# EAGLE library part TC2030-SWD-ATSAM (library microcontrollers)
TAG-CONNECT ICSP Connector Manufacturer: Tag-Connect Cable for easy In-Circuit Serial Programming. Designed for Microchip ICD2, suitable for many others. Two variants - one "with legs" (for hands-free fit on PCB) and another "without legs" for quick programming. PADDescription 1MCLR/Vpp 2Vdd 3GND 4PGD (ISPDAT) 5PGC (ISPCLK) 6nc (used for LVP) ©2009 ROFA.cz - modified and updated by Robert Darlington &#8249;rdarlington@gmail.com&#8250;
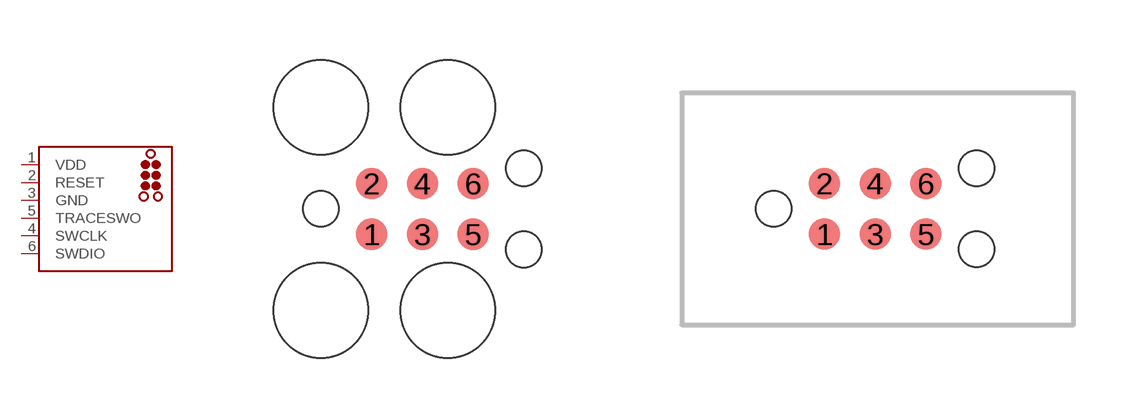
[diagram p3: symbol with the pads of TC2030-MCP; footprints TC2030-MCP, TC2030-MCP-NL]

Designator prefix J

## TC2030-SWD-ATSAM-MCP  [TC2030-MCP]
1  VDD  pwr
2  RESET  pwr
3  GND  pwr
4  SWCLK  in
5  TRACESWO  pwr
6  SWDIO

## TC2030-SWD-ATSAM-MCP-NL  [TC2030-MCP-NL]
Pads as for TC2030-MCP

## TC2030-SWD-ATSAM  [TC2030-MCP-NL-CP]
Pads as for TC2030-MCP

## Footprint TC2030-MCP (pad centres in mm)
TAG-CONNECT ICSP Connector - Legged version Manufacturer: Tag-Connect Cable for easy In-Circuit Serial Programming. Designed for Microchip ICD2, suitable for many others. NOTE: Eagle's default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
smd 0.787 x 0.787: 1 1.27,-0.635; 2 1.27,0.635; 3 2.54,-0.635; 4 2.54,0.635; 5 3.81,-0.635; 6 3.81,0.635
hole 0.889 at 0,0
hole 0.889 at 5.08,-1.016
hole 0.889 at 5.08,1.016
hole 2.375 at 0,2.54
hole 2.375 at 0,-2.54
hole 2.375 at 3.175,-2.54
hole 2.375 at 3.175,2.54

## Footprint TC2030-MCP-NL (pad centres in mm)
TAG-CONNECT ICSP Connector Manufacturer: Tag-Connect Cable for easy In-Circuit Serial Programming. Designed for Microchip ICD2, suitable for many others. PADDescription 1MCLR/Vpp 2Vdd 3GND 4PGD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
smd 0.787 x 0.787: 1 1.27,-0.635; 2 1.27,0.635; 3 2.54,-0.635; 4 2.54,0.635; 5 3.81,-0.635; 6 3.81,0.635
hole 0.889 at 0,0
hole 0.889 at 5.08,-1.016
hole 0.889 at 5.08,1.016

## Footprint TC2030-MCP-NL-CP (pad centres in mm)
TAG-CONNECT ICSP Connector- with optional copper pads for steel alignment pins Manufacturer: Tag-Connect Cable for easy In-Circuit Serial Programming. Designed for Microchip ICD2, suitable for many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
smd 0.787 x 0.787: 1 1.27,-0.635; 2 1.27,0.635; 3 2.54,-0.635; 4 2.54,0.635; 5 3.81,-0.635; 6 3.81,0.635
hole 1.6 at 0,0
hole 1.6 at 5.08,1.016
hole 1.6 at 5.08,-1.016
